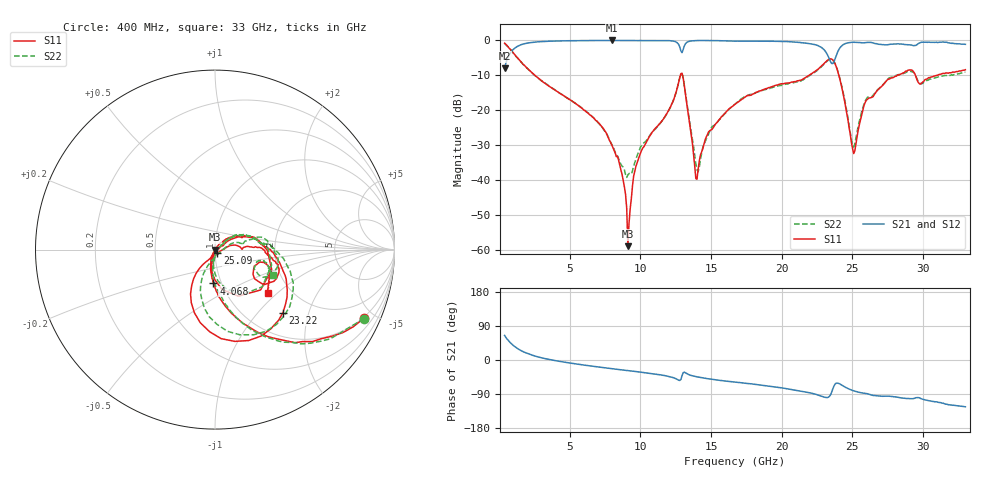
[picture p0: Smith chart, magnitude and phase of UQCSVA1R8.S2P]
!  Part Number  UQCSVA1R8  Mounting Orientation: Horizontal
!  Description: Ultra Low ESR Microwave capacitors
!  Application: Coupling, Bypass, Tuning, DC Block
!  Filters, Matching
# GHZ S DB R 50
! Freq  |S11|  S11 Ph  |S21|  S21 Ph  |S12|  S12 Ph  |S22|  S22 Ph
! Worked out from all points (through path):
!   401 points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, 400 MHz to 33 GHz, reference 50 ohm
!   highest |S21| = 0.00 dB at 7.98 GHz (marker M1); lowest = -7.9 dB at 400 MHz (marker M2)
!   group delay of S21, straight-line fit = 11.8 ps
!   lowest |S11| = -58.9 dB at 9.121 GHz (marker M3), VSWR 1.00, Z = 50.1 - j0.0925 ohm
!   |S11| at or under -10 dB: 2.546 GHz to 12.84 GHz (10.29 GHz wide, 134 % of centre); 12.99 GHz to 21.93 GHz (8.938 GHz wide, 51.2 % of centre); 24.05 GHz to 28.17 GHz (4.124 GHz wide, 15.8 % of centre)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
!   |S22| runs from -39.2 to -0.8 dB; largest |S21 - S12| = 0.017
!   S11 on the Smith chart (normalised r, x): 400 MHz: 0.94, -4.35; 4.068 GHz: 0.92, -0.36; 23.22 GHz: 1.44, -1.38; 25.09 GHz: 1.03, -0.04; 33 GHz: 1.54, -0.87
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0.4  -0.79 -24.8  -7.93 64.8  -7.94 64.7  -0.76 -24.8
1.704  -6.84 -67.6  -1.06 22.2  -1.06 21.8  -6.83 -67.8
4.068  -14.49 -92.5  -0.16 -2.2  -0.17 -2.3  -14.44 -90.7
5.861  -19.37 -103.1  -0.04 -12.5  -0.05 -12.5  -19.30 -96.7
7.98  -29.88 -115.6  0.00 -22.8  -0.01 -22.8  -29.75 -91.1
8.632  -37.13 -111.6  -0.01 -25.9  0.00 -26.0  -35.47 -73.1
9.121  -58.89 -54.4  -0.01 -28.1  -0.02 -28.1  -38.50 -22.7
9.854  -34.05 54.3  -0.01 -31.3  -0.01 -31.3  -32.13 31.5
11.321  -24.01 45.7  -0.01 -38.6  0.00 -38.6  -24.16 39.2
12.544  -14.70 24.8  -0.47 -49.8  -0.48 -49.8  -14.66 25.3
12.951  -9.39 -41.5  -3.49 -41.6  -3.44 -41.6  -9.50 -38.3
13.277  -17.80 -97.3  -0.58 -35.5  -0.60 -35.7  -17.40 -89.8
14.011  -39.72 -23.0  -0.03 -44.4  -0.04 -44.3  -37.08 -45.0
14.744  -27.01 27.3  -0.02 -49.2  -0.02 -49.0  -27.58 33.7
16.7  -18.29 31.1  -0.17 -58.3  -0.15 -58.3  -18.23 36.6
22.161  -9.42 -6.3  -1.06 -87.9  -1.06 -87.8  -9.55 0.5
23.22  -5.74 -42.8  -3.95 -99.3  -3.97 -98.8  -5.91 -32.1
23.954  -8.63 -108.1  -3.38 -60.9  -3.40 -61.0  -8.53 -95.1
25.095  -32.38 -55.9  -0.52 -81.3  -0.55 -81.0  -30.53 -42.2
25.991  -17.11 6.4  -0.61 -88.4  -0.64 -88.2  -16.74 14.1
27.621  -11.04 -3.2  -1.14 -95.6  -1.17 -95.4  -10.71 10.6
33  -8.37 -39.4  -1.11 -123.4  -1.13 -123.2  -9.09 -23.6
